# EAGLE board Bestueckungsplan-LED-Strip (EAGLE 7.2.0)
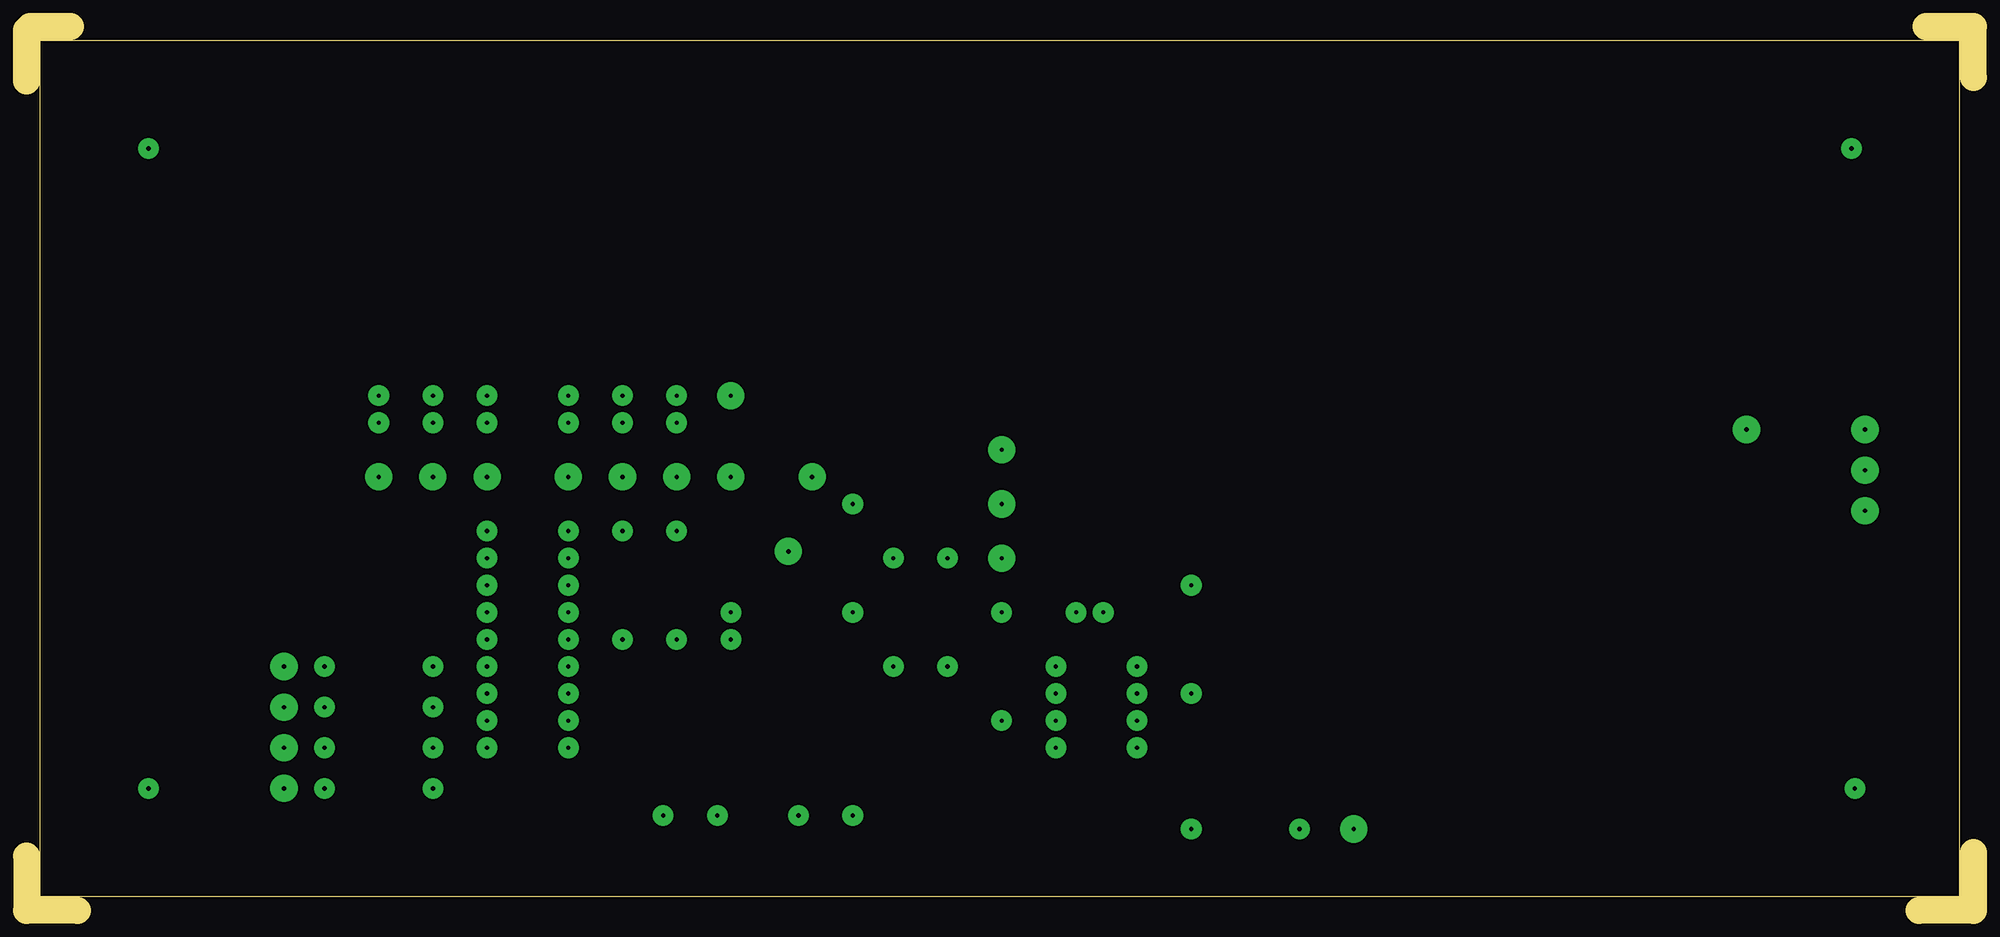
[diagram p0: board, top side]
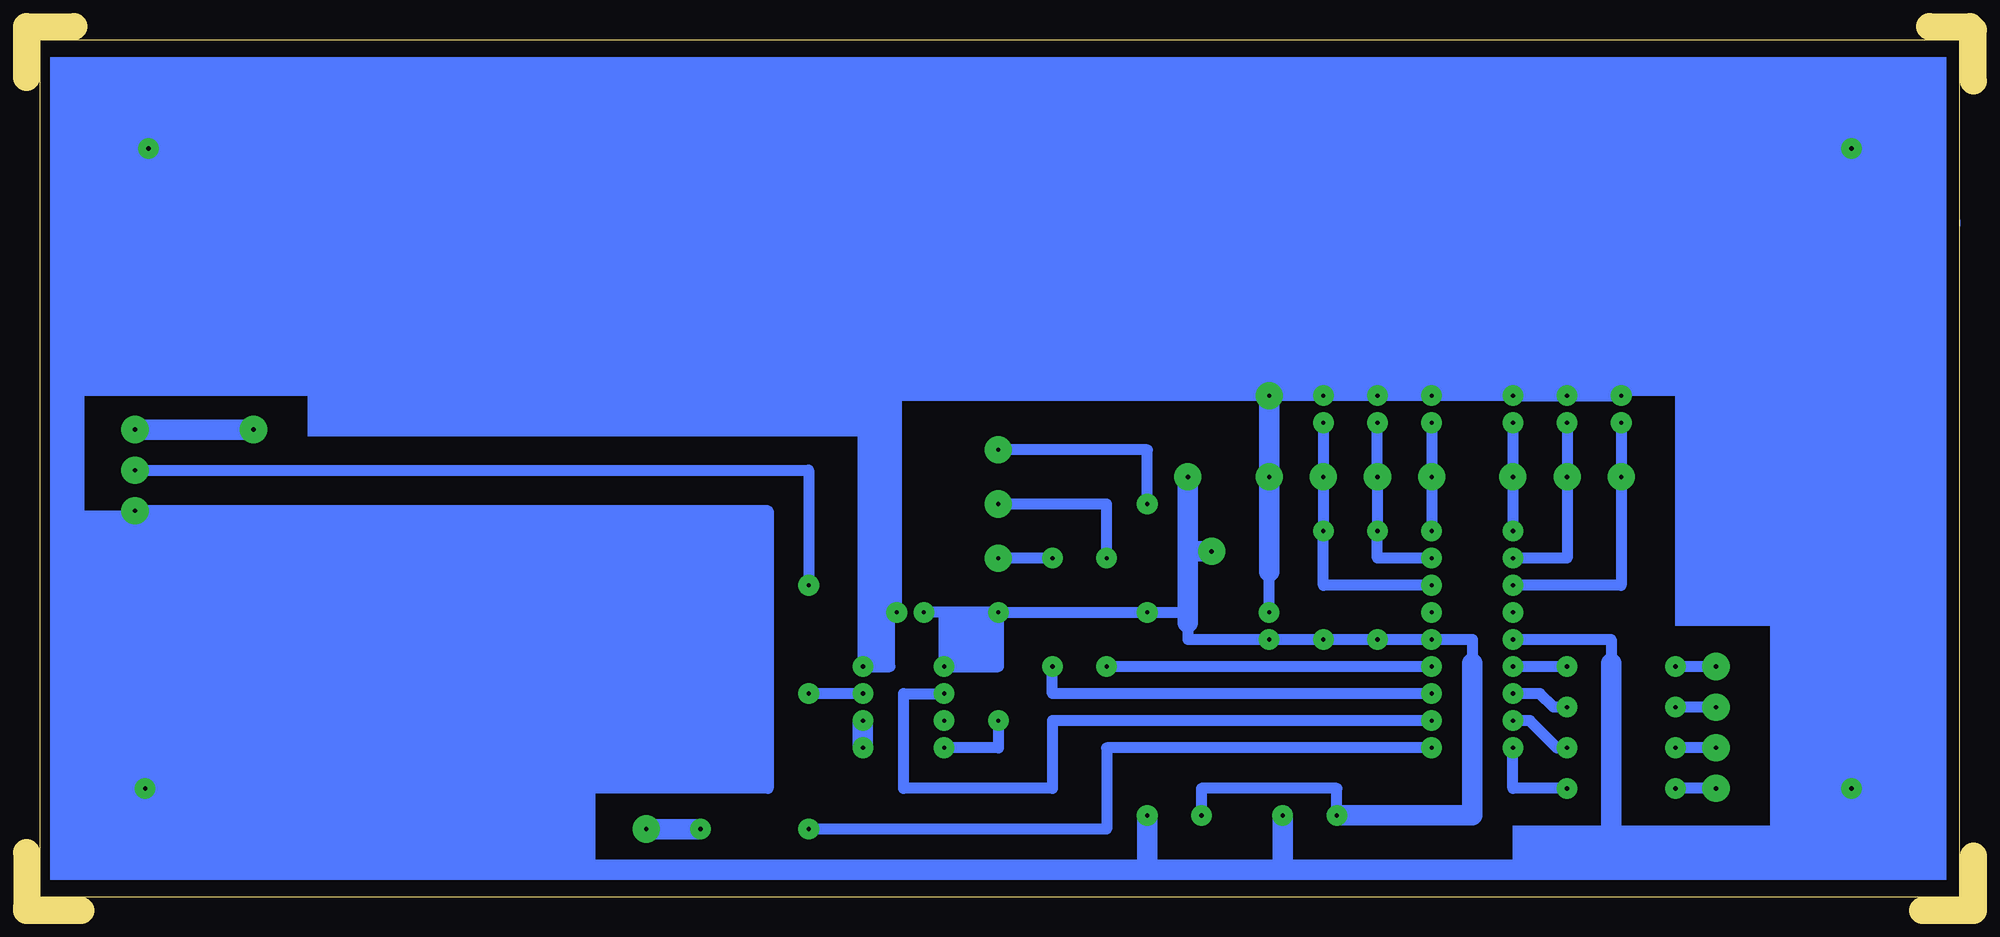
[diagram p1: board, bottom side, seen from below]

Size 182.56 x 82.87 mm. Coordinates in mm from the lower left corner, seen from the top.
Outline: 182.56,5.4 182.56,0.32
Outline: 182.56,0 177.48,0
Outline: 182.56,78.1 182.56,82.87 178.12,82.87
Outline: 0,5.08 0,0 4.76,0
Outline: 4.13,82.87 0.32,82.87
Outline: 0,77.79 0,82.55
Outline: 181.29,1.27 181.29,81.6 1.27,81.6 1.27,1.27 181.29,1.27
Copper layers (1*16): Top 0.035mm / dielectric 1.5mm / Bottom 0.035mm
Design rules "default": minimum track width 10mil, minimum drill 24mil, track to track 8mil, track to pad 8mil, pad to pad 8mil, via to via 8mil, smd to smd 8mil, copper to edge 40mil, drill to drill 8mil, minimum pad ring 10mil, minimum via ring 8mil, stop-mask expansion 4mil, vias tented up to drill 0mil, thermal gap 10mil

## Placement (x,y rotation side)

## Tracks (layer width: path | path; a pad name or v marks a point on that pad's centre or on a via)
S$1
  Bottom 1.016: 172.72,41.28 109.22,41.28 109.22,30.16
S$2  (via drill 0.4 pad 1.93)
  Bottom 1.016: v104.14,22.86 101.6,22.86 101.6,28.26
S$3  (via drill 0.4 pad 1.93, 0.4 pad 2.54)
  Bottom 1.016: 73.66,27.94 v77.47,27.94 v91.44,27.94 91.44,22.86 v96.52,22.86 96.52,27.94 | 73.66,27.94 73.66,26.99 73.66,25.4 v66.04,25.4 v60.96,25.4 v55.88,25.4 v50.8,25.4 46.99,25.4 46.99,23.18 | v59.69,8.89 59.69,11.43 72.39,11.43 v72.39,8.89 | v73.66,40.64 73.66,33.66 73.66,27.94 | 91.76,27.94 96.52,27.94 | 96.52,27.94 98.74,27.94
  Bottom 1.93: v71.44,33.66 73.66,33.66 | v59.69,8.89 46.99,8.89 46.99,23.18 | v73.66,40.64 73.66,26.99
S$4  (via drill 0.4 pad 1.93)
  other vias: 171.13,71.44
S$6
  Bottom 0: 1.27,64.77 1.27,64.14
S$10  (via drill 0.4 pad 1.93)
  other vias: 171.45,11.43
S$12  (via drill 0.4 pad 1.93)
  other vias: 11.43,11.43
S$13  (via drill 0.4 pad 1.93)
  Bottom 1.016: v50.8,22.86 v81.28,22.86
S$14  (via drill 0.4 pad 1.93)
  other vias: 109.22,20.32
S$15  (via drill 0.4 pad 1.93)
  Bottom 1.016: v38.1,22.86 v43.18,22.86
S$19  (via drill 0.4 pad 1.93)
  other vias: 43.18,27.94
S$22  (via drill 0.4 pad 1.93)
  other vias: 11.43,71.44
S$23  (via drill 0.4 pad 1.93)
  other vias: 109.22,30.48
S$29  (via drill 0.4 pad 1.93)
  other vias: 98.42,27.94
S$30  (via drill 0.4 pad 2.54)
  Bottom 1.93: v172.4,45.09 v161.29,45.09
S$32  (via drill 0.4 pad 1.93, 0.4 pad 2.54)
  Bottom 1.016: v77.47,38.1 77.47,43.18 v91.44,43.18
S$34  (via drill 0.4 pad 1.93)
  Bottom 1.016: v50.8,15.24 81.28,15.24 81.28,7.62 v109.22,7.62
S$35  (via drill 0.4 pad 1.93)
  Bottom 1.016: v38.1,19.05 39.37,19.05 40.64,20.32 v43.18,20.32
S$36  (via drill 0.4 pad 2.54)
  other vias: 172.4,41.28
S$37  (via drill 0.4 pad 1.93, 0.4 pad 2.54)
  Bottom 1.016: v43.18,25.4 33.97,25.4 33.97,23.18 | 33.97,4.76 33.97,3.81 64.77,3.81 77.47,3.81 137.16,3.81 137.16,11.43 | 137.16,11.43 113.03,11.43 113.03,37.47 | 137.16,11.43 113.03,37.47 | 113.03,37.47 v172.4,37.47
  Bottom 1.93: v64.77,8.89 64.77,3.81 | v77.47,8.89 77.47,3.81 | 33.97,4.76 33.97,23.18
S$39  (via drill 0.4 pad 1.93)
  Bottom 1.016: v50.8,17.78 86.36,17.78 86.36,11.43 100.33,11.43 100.33,20.32 v96.52,20.32
S$40  (via drill 0.4 pad 1.93)
  other vias: 50.8,27.94
S$43  (via drill 0.4 pad 1.93, 0.4 pad 2.54)
  Bottom 1.016: 25.08,22.86 v24.13,22.86 v27.94,22.86
S$44  (via drill 0.4 pad 1.93)
  other vias: 50.8,35.56
S$45  (via drill 0.4 pad 1.93)
  Bottom 1.93: v104.14,17.78 v104.14,15.24
S$46  (via drill 0.4 pad 1.93)
  Bottom 1.016: v38.1,15.24 39.05,15.24 41.59,17.78 v43.18,17.78
S$47  (via drill 0.4 pad 1.93)
  other vias: 104.14,20.32
S$48  (via drill 0.4 pad 1.93)
  Bottom 1.016: v38.1,11.43 43.18,11.43 v43.18,15.24
S$49  (via drill 0.4 pad 1.93)
  other vias: 96.52,17.78
S$50
  Bottom 1.016: 104.46,20.32 109.22,20.32
S$52  (via drill 0.4 pad 1.93, 0.4 pad 2.54)
  Bottom 1.016: v24.13,19.05 v27.94,19.05
S$53  (via drill 0.4 pad 1.93, 0.4 pad 2.54)
  Bottom 1.016: v81.28,33.02 81.28,38.1 v91.44,38.1
S$54  (via drill 0.4 pad 1.93, 0.4 pad 2.54)
  Bottom 1.016: v86.36,33.02 v91.44,33.02
S$56  (via drill 0.4 pad 1.93)
  Bottom 1.016: v91.44,17.78 91.44,15.24 v96.52,15.24
S$58  (via drill 0.4 pad 1.93, 0.4 pad 2.54)
  Bottom 1.93: v119.38,7.62 v124.46,7.62
S$59  (via drill 0.4 pad 1.93, 0.4 pad 2.54)
  Bottom 1.016: v24.13,15.24 v27.94,15.24
S$63  (via drill 0.4 pad 1.93, 0.4 pad 2.54)
  Bottom 1.016: v24.13,11.43 v27.94,11.43
S$68  (via drill 0.4 pad 1.93, 0.4 pad 2.54)
  Bottom 1.016: v50.8,33.02 55.88,33.02 v55.88,35.56 v55.88,40.64 v55.88,45.72
S$70  (via drill 0.4 pad 1.93)
  Bottom 1.016: v50.8,20.32 86.36,20.32 v86.36,22.86
S$71  (via drill 0.4 pad 1.93, 0.4 pad 2.54)
  Bottom 1.016: v50.8,30.48 60.96,30.48 v60.96,35.56 v60.96,40.64 v60.96,45.72
S$72  (via drill 0.4 pad 2.54)
  other vias: 50.8,40.64
S$74  (via drill 0.4 pad 1.93)
  Bottom 1.016: v50.8,45.72 50.8,35.24
S$76  (via drill 0.4 pad 2.54)
  other vias: 43.18,40.64
S$77  (via drill 0.4 pad 2.54)
  other vias: 38.1,40.64
S$78  (via drill 0.4 pad 2.54)
  other vias: 33.02,40.64
S$80  (via drill 0.4 pad 1.93)
  Bottom 1.016: v43.18,45.72 v43.18,35.56
S$82  (via drill 0.4 pad 1.93, 0.4 pad 2.54)
  Bottom 1.016: v66.04,27.94 66.04,31.75 v66.04,40.64 v66.04,48.26 | v66.04,48.26 104.14,48.26 104.14,27.94 | 104.14,27.94 v100.96,27.94 100.96,48.9 | 104.14,27.94 104.14,22.54 | v66.04,48.26 v60.96,48.26 v55.88,48.26 v50.8,48.26 v43.18,48.26 v33.02,48.26
  Bottom 1.93: v66.04,48.26 66.04,31.75
S$83  (via drill 0.4 pad 1.93)
  Bottom 1.016: v38.1,45.72 38.1,33.02 v43.18,33.02
S$84  (via drill 0.4 pad 1.93)
  other vias: 38.1,48.26
S$85  (via drill 0.4 pad 1.93)
  Bottom 1.016: v33.02,45.72 33.02,30.48 v43.18,30.48
(copper drawn outside any net)
  shapes: Bottom area x15

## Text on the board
Vias: Auf Bestückungsseite gesehen !
Dimension: 1 stck. Anschluss-Leiste 1,2mm
tOrigins: PIC16F1827 | PIC12F1840 | 1 | Links oben ist | immer PIN 1 | LED rot/gelb/grün/blau | Taster vorw. | Taster rückw. | Poti rt | Poti gn | Poti Tempo | +5V Schalter | +5Volt Stromversorgung | 47n | 47n | 47n | 47n | 47n | 47n | LED gn Kontrolle | Poti bl | +5V Schalter | Masse | Datenleitung | LED gl Tempo | -Pol Stromversorgung | 1 | Masse | +5V | LED bl Farbe | 470 | 47n | 470 | 10K | 10K | 47n | Katode | 1K | 470 | 1 | Anode | LED rt | 1K | immer an + Pol | 10K | LED rt | 1K | PIC16F1827 | LED rt | 1K | PIC12F1840 | LED rt | 1K | 2mal 470µ/25V | LED rt | + | 1K | + | BOHRUNGEN | alles 0.8mm vorbohren | Leiterplatte: | 4 stck. Befestigungsbohr... 3,2mm | 1,5mm dick | Cevausit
